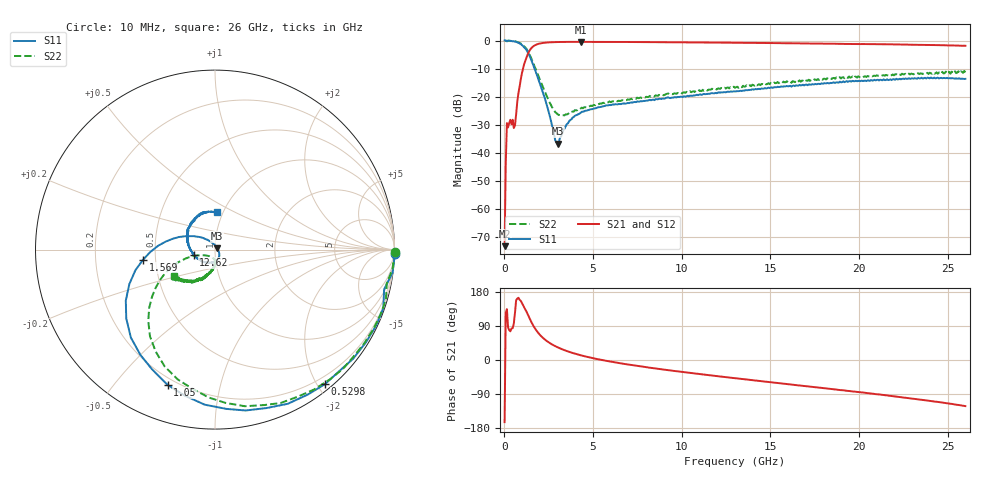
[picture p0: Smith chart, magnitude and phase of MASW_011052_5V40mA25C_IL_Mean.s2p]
! MA-COM, USA
! Part Number: MASW-011052
! Data: 29-03-2013
! Bias Condition:
!  Insertion Loss in ON stage Antenna (1) to RFin (2)
!  Forward Bias (series Diode and Shunt Diode) I = 40 mA
!  Reverse Bias Voltage V = -5V
!  Temp: 25C
!  VAR RecID: Mean
# HZ S DB R 50
! F n11x n11y n21x n21y n12x n12y n22x n22y
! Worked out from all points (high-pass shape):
!   401 points, 10 MHz to 26 GHz, reference 50 ohm
!   highest |S21| = -0.47 dB at 4.298 GHz (marker M1); lowest = -73.3 dB at 10 MHz (marker M2)
!   |S21| within 3 dB of the highest: 1.43 GHz to end of sweep
!   lowest |S11| = -36.8 dB at 2.999 GHz (marker M3), VSWR 1.03, Z = 51.3 + j0.659 ohm
!   |S11| at or under -10 dB: 1.7 GHz to end of sweep
!   |S22| runs from -26.8 to 0.0 dB; largest |S21 - S12| = 0.013
!   S11 on the Smith chart (normalised r, x): 10 MHz: -11, -89; 529.8 MHz: 0.09, -2.11; 1.05 GHz: 0.17, -0.70; 1.569 GHz: 0.42, -0.06; 12.62 GHz: 0.79, -0.05; 26 GHz: 0.94, +0.41
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1e7  0.02 -1.3  -73.33 -164.0  -77.61 -175.8  0.00 -0.8
2.0493e8  -0.06 -19.3  -31.00 86.0  -31.05 86.0  -0.06 -16.2
2.699e8  -0.07 -25.4  -29.39 78.7  -29.43 78.7  -0.09 -21.4
5.298e8  -0.28 -50.7  -31.21 96.3  -31.24 96.5  -0.22 -42.9
6.5975e8  -0.45 -64.7  -26.35 157.8  -26.37 158.0  -0.40 -54.6
7.897e8  -0.80 -79.2  -18.74 164.2  -18.76 164.4  -0.63 -66.8
1.0496e9  -1.95 -109.3  -10.07 145.1  -10.08 145.3  -1.67 -92.4
1.3095e9  -4.07 -142.2  -4.95 121.0  -4.94 121.2  -3.64 -120.1
1.5694e9  -7.82 -171.8  -2.39 95.5  -2.38 95.5  -7.17 -143.2
1.8293e9  -12.25 165.8  -1.37 76.1  -1.36 76.2  -11.26 -157.2
2.2192e9  -19.46 139.4  -0.82 56.5  -0.82 56.6  -17.30 -163.5
2.8039e9  -33.64 80.8  -0.57 38.0  -0.58 38.0  -24.89 -143.7
2.9989e9  -36.77 26.3  -0.54 33.5  -0.54 33.5  -26.28 -131.0
3.5836e9  -29.52 -46.8  -0.49 22.6  -0.50 22.6  -26.22 -99.7
4.2984e9  -25.80 -68.7  -0.47 12.6  -0.48 12.6  -24.24 -87.3
4.3633e9  -25.39 -68.5  -0.47 11.7  -0.48 11.8  -23.94 -89.4
8.7167e9  -20.77 -130.4  -0.59 -23.6  -0.60 -23.5  -19.39 -94.6
1.2615e10  -18.21 -165.9  -0.78 -45.9  -0.78 -45.8  -16.74 -106.9
1.3005e10  -18.16 -168.0  -0.80 -48.0  -0.79 -47.9  -16.86 -107.9
1.7358e10  -15.57 158.6  -1.06 -70.8  -1.09 -70.7  -13.94 -121.4
2.1712e10  -13.98 127.5  -1.36 -94.3  -1.36 -94.0  -12.18 -133.7
2.6e10  -13.67 86.3  -1.88 -121.7  -1.93 -121.2  -11.38 -147.7
